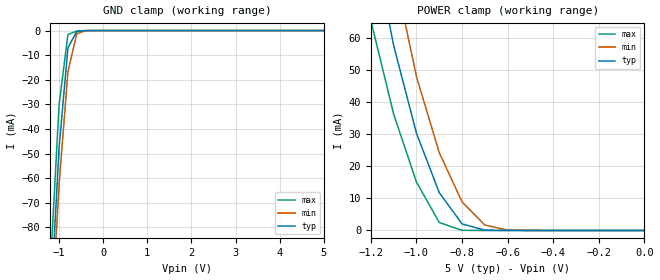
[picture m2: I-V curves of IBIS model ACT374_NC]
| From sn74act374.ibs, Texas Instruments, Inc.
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|   Model ACT374_NC
[Model]   ACT374_NC
Model_type  Input
Polarity   Non-Inverting
Vinl = 0.8
Vinh = 2.0
| variable   typ   min   max
C_comp   2.5pF   NA   NA
[Temperature Range]   40   100   -40
| Ambient temperature   25   85   -40
[Voltage range]   5.0   4.5   5.5
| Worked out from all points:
|   GND clamp passes 1 mA (typ) near -0.62 V on its own axis
|   POWER clamp passes 1 mA (typ) near -0.75 V on its own axis
[GND Clamp]
|   Voltage   I(typ)   I(min)   I(max)
-5V       -1.865A    -1.667A    -2.091A
-1.2V     -114.1mA   -125.6mA   -96.94mA
-1V       -47.54mA   -62.5mA    -30.14mA
-800mV    -7.006mA   -16.76mA   -1.613mA
-600mV    -351.8uA   -1.289mA   -203.9uA
-400mV    -14.77uA   -55.28uA   -1.425uA
5V        104.2pA    153.3pA    26.02pA
[POWER Clamp]
|   Voltage   I(typ)   I(min)   I(max)
-5V       2.866A     2.324A     3.957A
-1.2V     94.02mA    118.2mA    65.37mA
-1.1V     57.62mA    81.54mA    36.25mA
-1V       30.31mA    47.95mA    15.1mA
-900mV    11.79mA    24.26mA    2.488mA
-800mV    2.057mA    8.907mA    43.58uA
-700mV    87.35uA    1.696mA    334.7nA
-600mV    1.937uA    125.8uA    2.515nA
0V        4.16pA     376.9pA    4.38pA
